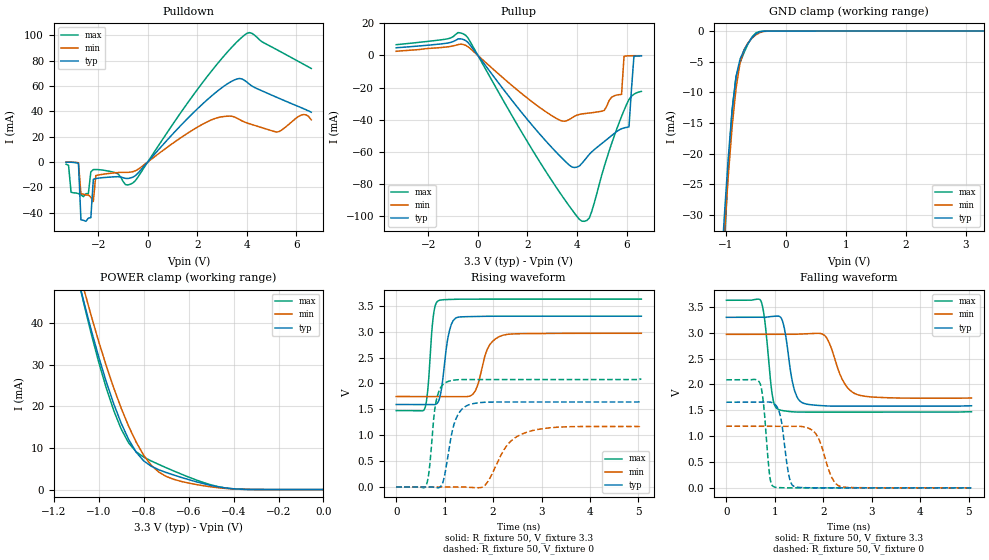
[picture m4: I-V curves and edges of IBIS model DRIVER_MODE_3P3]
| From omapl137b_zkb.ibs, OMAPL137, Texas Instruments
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|   Model Cell DRIVER_MODE_3P3
|DRIVER_MODE_3P3
[Model]   DRIVER_MODE_3P3
Model_type   I/O
Polarity   Non-Inverting
Enable   Active-Low
Vinl =  0.8
Vinh =  2
Cref =  15.0000pF
Rref =  100.0000M
Vref =  0V
Vmeas =  1.65
C_comp   1.652921p   1.424215p   1.79759p
[Model Spec]
Vinl   0.8   0.8   0.8
Vinh   2   2   2
[Temperature Range]   25   125   -40
[Voltage Range]   3.3   2.97   3.63
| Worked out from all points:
|   slope of the pulldown table from 0 to 0.495 V, typ, clamps not added: 45 ohm
|   slope of the pullup table from 0 to 0.495 V, typ, clamps not added: 48.5 ohm
|   GND clamp passes 1 mA (typ) near -0.56 V on its own axis
|   POWER clamp passes 1 mA (typ) near -0.50 V on its own axis
|   rising waveform, R_fixture 50, V_fixture 3.3: 20-80 % time 142ps typ, 228ps min, 98.5ps max; typ from 1.59 V to 3.3 V
|   rising waveform, R_fixture 50, V_fixture 0: 20-80 % time 214ps typ, 466ps min, 135ps max; typ from 0 V to 1.65 V
|   falling waveform, R_fixture 50, V_fixture 3.3: 20-80 % time 171ps typ, 306ps min, 134ps max; typ from 3.3 V to 1.59 V
|   falling waveform, R_fixture 50, V_fixture 0: 20-80 % time 143ps typ, 254ps min, 111ps max; typ from 1.66 V to 0 V
| Nom Voltages:
|   VDD=1, VDDS=3.3, VSS=0, VSSS=0
| Min Voltages:
|   VDD=0.99, VDDS=2.97, VSS=0, VSSS=0
| Max Voltages:
|   VDD=1.21, VDDS=3.63, VSS=0, VSSS=0
[POWER_clamp]
|   voltage   I(typ)   I(min)   I(max)
-3.3V     637.1mA    797mA      659.4mA
-1.1V     52.42mA    55.11mA    52.45mA
-1.067V   45.17mA    48.25mA    44.73mA
-1.033V   38.29mA    41.71mA    37.39mA
-966.7mV  25.92mA    29.76mA    24.4mA
-900mV    15.92mA    19.54mA    14.52mA
-833.3mV  8.978mA    11.39mA    9.072mA
-800mV    6.903mA    8.251mA    7.811mA
-733.3mV  4.783mA    4.233mA    6.06mA
-633.3mV  2.943mA    1.978mA    3.735mA
-433.3mV  380.5uA    277.9uA    364.2uA
0V        11.23uA    4.832uA    22.77uA
[Pulldown]
|   voltage   I(typ)   I(min)   I(max)
-3.3V     -207uA     -143.1uA   -1.781mA
-3.1V     -258.6uA   -179.5uA   -23.88mA
-2.8V     -1.162mA   -653.7uA   -25.03mA
-2.7V     -45.72mA   -25.09mA   -26.01mA
-2.5V     -46.87mA   -26.19mA   -25.09mA
-2.3V     -44.01mA   -27.87mA   -7.781mA
-2.2V     -13.77mA   -31.25mA   -6.063mA
-2.1V     -13.16mA   -10.74mA   -6.007mA
-500mV    -10.82mA   -7.008mA   -14.76mA
2.6V      52.45mA    33.42mA    72.37mA
4V        63.02mA    30.81mA    101.4mA
6.6V      39.22mA    33.23mA    73.74mA
[Pullup]
|   voltage   I(typ)   I(min)   I(max)
-3.3V     4.784mA    2.583mA    6.695mA
-500mV    9.328mA    6.329mA    12.63mA
3.1V      -59.14mA   -38.53mA   -80.53mA
3.8V      -69.36mA   -38.73mA   -95.99mA
4.2V      -67.05mA   -36.35mA   -103mA
4.5V      -61.45mA   -35.78mA   -101mA
5.1V      -53.53mA   -34.18mA   -69.08mA
5.8V      -45.54mA   -24.19mA   -37.93mA
5.9V      -45.04mA   -477.7uA   -34.14mA
6.1V      -44.38mA   -204.6uA   -27.37mA
6.3V      -522.4uA   -151.8uA   -24.08mA
6.6V      -227uA     -145.4uA   -22.35mA
[GND_clamp]
|   voltage   I(typ)   I(min)   I(max)
-3.3V     -540.4mA   -632.1mA   -650mA
-1.1V     -42.19mA   -44.77mA   -50.4mA
-1.033V   -30.93mA   -33.9mA    -36.08mA
-966.7mV  -21.12mA   -24.1mA    -23.15mA
-900mV    -13.04mA   -15.76mA   -12.95mA
-833.3mV  -7.421mA   -9.341mA   -7.462mA
-766.7mV  -4.587mA   -5.19mA    -5.139mA
-700mV    -3.115mA   -3.042mA   -3.512mA
-566.7mV  -1.077mA   -1.16mA    -951.8uA
-500mV    -427.2uA   -595.8uA   -282.5uA
-233.3mV  -323.2nA   -2.802uA   -126.6nA
3.3V      19.7uA     43.77uA    39.19uA
[Ramp]
| variable   typ   min   max
dV/dt_f  1.1129735/0.1423253n 0.78701463/0.27485677n  1.3857564/87.193476p
dV/dt_r  1.0364073/0.18498376n 0.73917937/0.41564114n  1.3085596/0.11643162n
R_load = 50
[Rising Waveform]
R_fixture = 50
V_fixture = 3.3
V_fixture_min = 2.97
V_fixture_max = 3.63
|   time   V(typ)   V(min)   V(max)
0s        1.595V     1.749V     1.476V
594.7ps   1.594V     1.748V     1.529V
768.8ps   1.591V     1.748V     3.322V
873.4ps   1.659V     1.748V     3.6V
1.09ns    2.985V     1.748V     3.623V
1.265ns   3.279V     1.747V     3.628V
1.604ns   3.294V     1.816V     3.63V
1.887ns   3.299V     2.677V     3.63V
2.2ns     3.3V       2.932V     3.63V
5.06ns    3.3V       2.97V      3.63V
[Rising Waveform]
R_fixture = 50
V_fixture = 0
V_fixture_min = 0
V_fixture_max = 0
|   time   V(typ)   V(min)   V(max)
0s        0V         0V         0V
616.8ps   0V         0V         29.54mV
827.6ps   -12.91mV   0V         1.674V
1.046ns   474.2mV    0V         2.03V
1.227ns   1.305V     0V         2.069V
1.518ns   1.594V     -6.83mV    2.076V
1.832ns   1.638V     33.64mV    2.076V
2.293ns   1.643V     814.3mV    2.077V
2.711ns   1.643V     1.065V     2.077V
5.06ns    1.649V     1.174V     2.085V
[Falling Waveform]
R_fixture = 50
V_fixture = 3.3
V_fixture_min = 2.97
V_fixture_max = 3.63
|   time   V(typ)   V(min)   V(max)
0s        3.3V       2.97V      3.63V
712.2ps   3.3V       2.97V      3.619V
945.5ps   3.317V     2.97V      1.813V
1.077ns   3.322V     2.97V      1.516V
1.195ns   3.103V     2.97V      1.49V
1.407ns   1.887V     2.971V     1.469V
1.56ns    1.651V     2.978V     1.466V
2.032ns   1.586V     2.947V     1.466V
2.7ns     1.581V     1.805V     1.466V
5.06ns    1.588V     1.739V     1.474V
[Falling Waveform]
R_fixture = 50
V_fixture = 0
V_fixture_min = 0
V_fixture_max = 0
|   time   V(typ)   V(min)   V(max)
0s        1.657V     1.192V     2.091V
698.3ps   1.657V     1.193V     2.016V
895ps     1.661V     1.192V     235.9mV
984.3ps   1.629V     1.192V     19.46mV
1.112ns   1.401V     1.192V     3.593mV
1.291ns   237.3mV    1.193V     0V
1.4ns     27.06mV    1.193V     0V
1.856ns   0V         1.035V     0V
2.347ns   0V         28.45mV    0V
5.06ns    0V         0V         0V
